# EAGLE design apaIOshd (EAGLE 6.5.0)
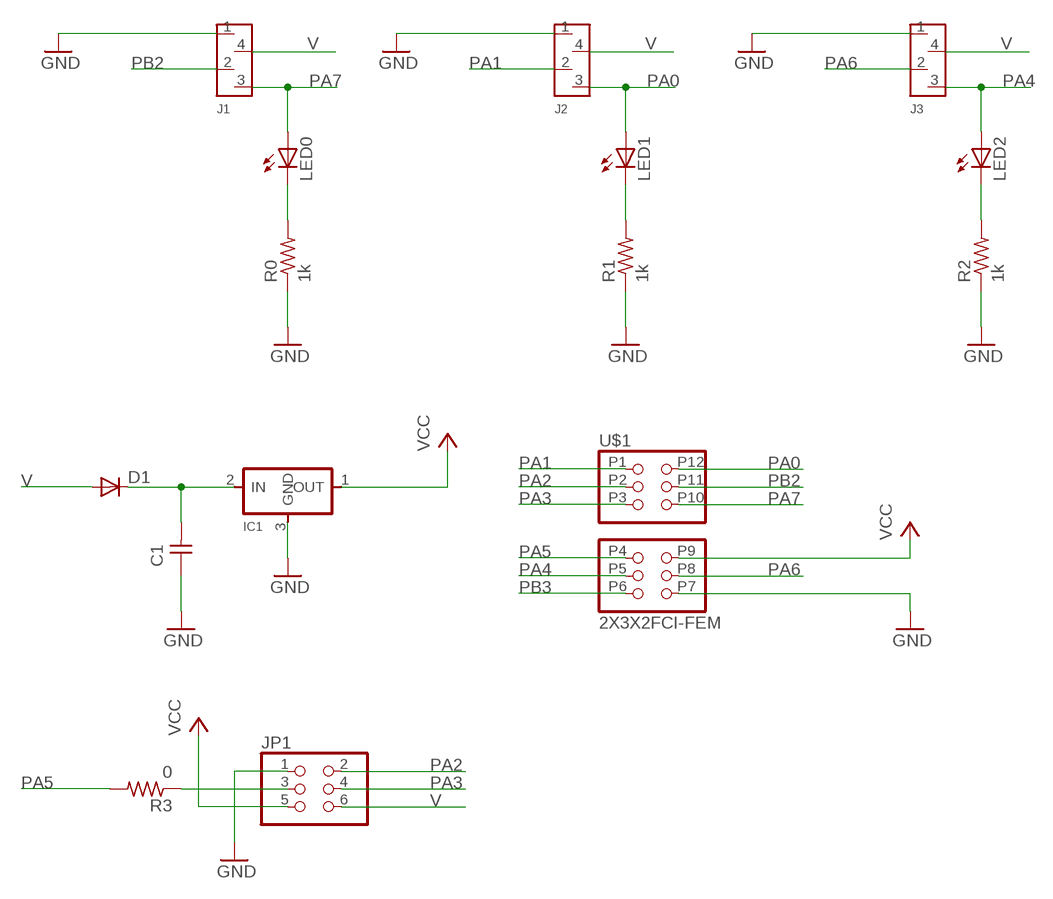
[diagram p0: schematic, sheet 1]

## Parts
C1  UNPOLARIZED_CAPACITOR1206  [1206]
D1  DIODESOD123  [SOD123]
IC1  REGULATORSOT23  [SOT23]
J1  APA 0  MTA_4MTA_4  [MTA_4]
J2  APA 1  MTA_4MTA_4  [MTA_4]
J3  APA 2  MTA_4MTA_4  [MTA_4]
JP1  PINHD-2X3-SMD  [2X03SMD]
LED0  LED1206  [1206]
LED1  LED1206  [1206]
LED2  LED1206  [1206]
R0  1k  RESISTOR1206  [1206]
R1  1k  RESISTOR1206  [1206]
R2  1k  RESISTOR1206  [1206]
R3  0  RESISTOR1206  [1206]
U$1  2X3X2FCI-FEM  [2X03X2FCI-FEM]

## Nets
GND: C1.1 IC1.3(GND) J1.1 J2.1 J3.1 JP1.1 R0.1 R1.1 R2.1 U$1.P7
N$1: C1.2 D1.CATHODE(C) IC1.2(IN)
N$2: JP1.3 R3.1
N$3: LED0.2(C) R0.2
N$5: LED1.2(C) R1.2
N$6: LED2.2(C) R2.2
PA0: J2.3 LED1.1(A) U$1.P12
PA1: J2.2 U$1.P1
PA2: JP1.2 U$1.P2
PA3: JP1.4 U$1.P3
PA4: J3.3 LED2.1(A) U$1.P5
PA5: R3.2 U$1.P4
PA6: J3.2 U$1.P8
PA7: J1.3 LED0.1(A) U$1.P10
PB2: J1.2 U$1.P11
PB3: U$1.P6
V: D1.ANODE(A) J1.4 J2.4 J3.4 JP1.6
VCC: IC1.1(OUT) JP1.5 U$1.P9

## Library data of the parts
C1 = 01_FAB_Hello:UNPOLARIZED_CAPACITOR: unpolarized_capacitor
D1 = 01_fab:DIODE: DIODE
IC1 = 01_fab:REGULATOR
J1-J3 = 01_ng:MTA_4
JP1 = 01_fab:PINHD-2X3-SMD: PIN HEADER
LED0 LED1 LED2 = 01_FAB_Hello:LED
R0 R1-R3 = 01_FAB_Hello:RESISTOR
U$1 = ot:2X3X2FCI-FEM: Use 2 FCI female headers as through hole components on PCB

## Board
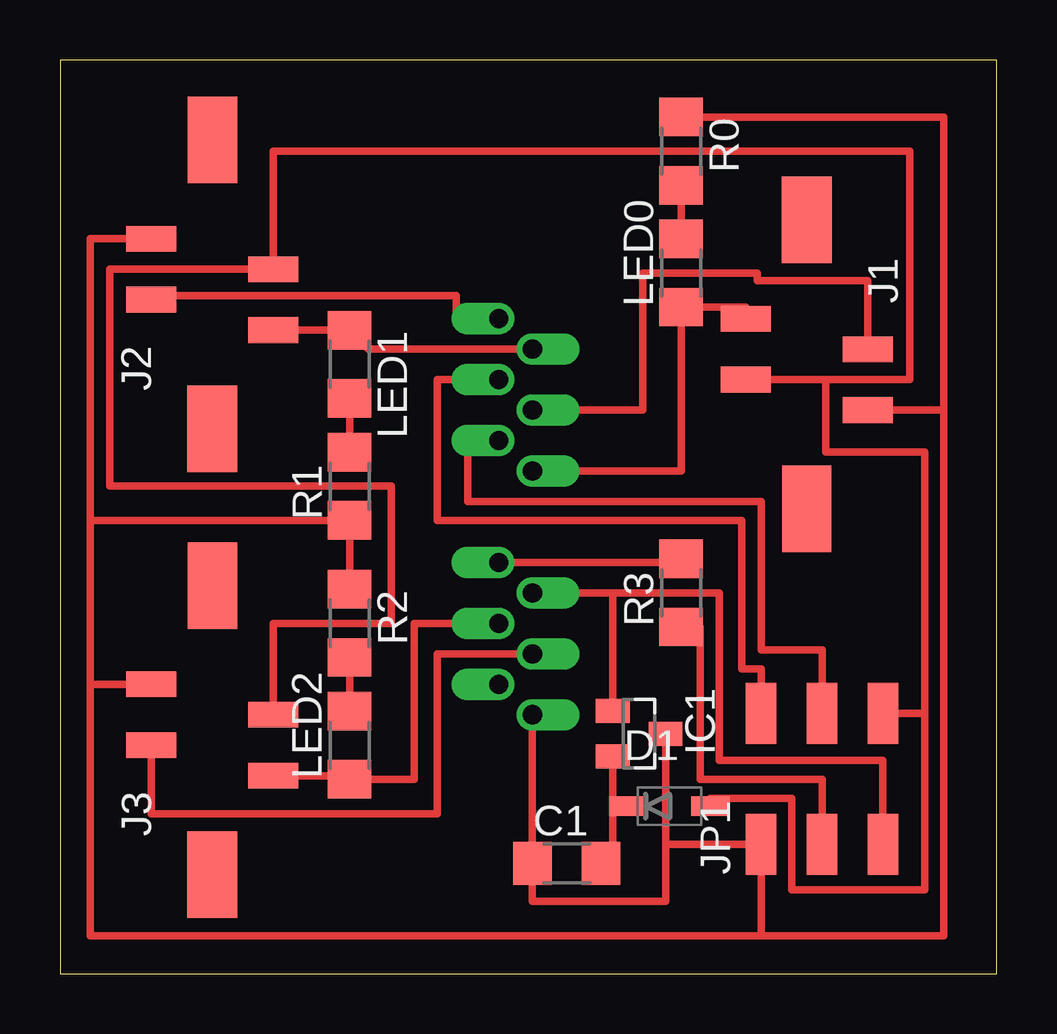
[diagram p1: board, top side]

Size 39.04 x 38.09 mm. Coordinates in mm from the lower left corner, seen from the top.
Outline: 0,0 39.04,0 39.04,38.09 0,38.09 0,0
Copper layers (1*16): Top 0.035mm / dielectric 1.5mm / Bottom 0.035mm
Design rules "default *": minimum track width 10mil, minimum drill 24mil, track to track 0.4mm, track to pad 0.4mm, pad to pad 0.4mm, via to via 0.4mm, smd to smd 0.4mm, copper to edge 40mil, drill to drill 8mil, minimum pad ring 10mil, minimum via ring 8mil, stop-mask expansion 4mil, vias tented up to drill 0mil, thermal gap 10mil

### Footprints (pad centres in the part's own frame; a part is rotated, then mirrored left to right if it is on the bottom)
1206 = smd 1.6 x 1.803: 1 -1.422,0; 2 1.422,0
SOD123 = smd 1.6 x 0.8: ANODE 1.7,0; CATHODE -1.7,0
SOT23 = smd 1 x 1.4: 1 -0.95,-1.1; 2 0.95,-1.1; 3 0,1.1
MTA_4 = smd 1.067 x 2.083: 1 -1.905,-2.54; 2 0.635,-2.54; 3 1.905,2.54; 4 -0.635,2.54 | smd 3.607 x 2.057: P$5 -6.02,0 | smd 3.607 x 2.083: P$6 6.02,0
2X03SMD = smd 2.54 x 1.27: 1 -2.54,2.54; 2 2.92,2.54; 3 -2.54,0; 4 2.92,0; 5 -2.54,-2.54; 6 2.92,-2.54
2X03X2FCI-FEM = drill 0.8 pad 1.27 offset: P1 3.045,18.415; P2 3.045,15.875; P3 3.045,13.335; P4 3.045,8.255; P5 3.045,5.715; P6 3.045,3.175; P7 4.445,1.905; P8 4.445,4.445; P9 4.445,6.985; P10 4.445,12.065; P11 4.445,14.605; P12 4.445,17.145

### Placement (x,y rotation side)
C1  21.11,4.6 0 top
D1  25.4,6.99 0 top
IC1  24.13,10 270 top
J1  31.11,25.4 90 top
J2  6.35,28.73 270 top
J3  6.35,10.16 270 top
JP1  31.75,7.94 90 top
LED0  25.88,29.21 90 top
LED1  12.06,25.4 270 top
LED2  12.06,9.53 90 top
R0  25.88,34.29 270 top
R1  12.06,20.32 90 top
R2  12.06,14.61 270 top
R3  25.88,15.88 90 top
U$1  15.24,8.89 0 top

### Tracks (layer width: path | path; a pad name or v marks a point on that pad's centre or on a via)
GND
  Top 0.305: J2.1 1.27,30.64 1.27,18.9 | 1.27,18.9 1.27,12.06 | 1.27,12.06 1.27,1.59 29.21,1.59 | 29.21,1.59 36.83,1.59 36.83,23.5 | 36.83,23.5 J1.1 | J3.1 1.27,12.06 | R0.1 36.83,35.71 36.83,23.5 | 1.27,18.9 R1.1 R2.1 | 29.21,1.59 JP1.1 25.23,5.4 | 25.23,5.4 IC1.3 | C1.1 U$1.P7 19.68,3.02 25.23,3.02 25.23,5.4
N$1
  Top 0.305: IC1.2 23.03,6.99 | 23.03,6.99 23.03,4.6 C1.2 | D1.CATHODE 23.03,6.99
N$2
  Top 0.305: JP1.3 31.75,8.1 26.67,8.1 26.67,14.45 R3.1
N$3
  Top 0.305: LED0.2 R0.2
N$5
  Top 0.305: R1.2 LED1.2
N$6
  Top 0.305: R2.2 LED2.2
PA0
  Top 0.305: U$1.P12 12.85,26.04 LED1.1 J2.3
PA1
  Top 0.305: U$1.P1 16.51,27.3 16.51,28.26 3.81,28.26 J2.2
PA2
  Top 0.305: JP1.2 29.21,12.7 28.42,12.7 28.42,18.89 15.72,18.89 15.72,24.77 U$1.P2
PA3
  Top 0.305: JP1.4 31.75,13.49 29.21,13.49 29.21,19.68 16.99,19.68 16.99,22.23 U$1.P3
PA4
  Top 0.305: J3.3 12.06,8.26 LED2.1 14.76,8.1 14.76,14.61 U$1.P5
PA5
  Top 0.305: U$1.P4 25.88,17.14 R3.2
PA6
  Top 0.305: J3.2 3.81,6.67 15.72,6.67 15.72,13.34 U$1.P8
PA7
  Top 0.305: J1.3 28.57,27.79 LED0.1 25.88,20.95 U$1.P10
PB2
  Top 0.305: J1.2 33.66,28.89 29.05,28.89 29.05,29.21 24.29,29.21 24.29,23.5 U$1.P11
V
  Top 0.305: J3.4 8.89,14.61 13.81,14.61 13.81,20.32 2.06,20.32 2.06,29.37 J2.4 8.89,34.29 35.4,34.29 35.4,24.77 31.91,24.77 | J1.4 31.91,24.77 | 36.04,10.86 36.04,3.49 30.48,3.49 30.48,7.3 27.1,7.3 D1.ANODE | 36.04,10.86 36.04,21.75 31.91,21.75 31.91,24.77 | JP1.6 36.04,10.86
VCC
  Top 0.305: JP1.5 34.29,8.89 27.46,8.89 27.46,15.88 23.03,15.88 | IC1.1 23.03,15.88 | 23.03,15.88 U$1.P9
